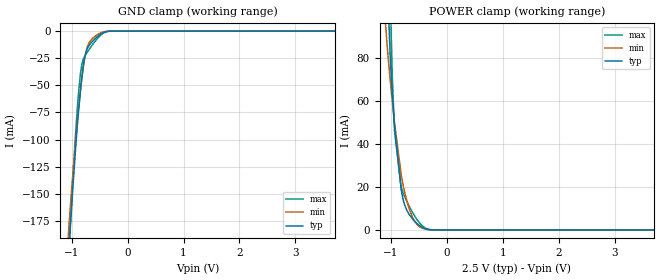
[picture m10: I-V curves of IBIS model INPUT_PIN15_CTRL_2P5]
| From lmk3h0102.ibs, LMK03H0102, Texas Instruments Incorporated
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[Model]   INPUT_PIN15_CTRL_2P5
Model_type   Input
Vinl = 0.4
Vinh = 1.625
|   typ   min   max
C_comp   0.7pF   0.5pF   0.9pF
[Voltage Range]   2.5   2.375   2.625
[Temperature Range]   45   125   -40
[Power Clamp Reference]   2.5   2.375   2.625
[GND Clamp Reference]   0   0   0
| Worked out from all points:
|   GND clamp passes 1 mA (typ) near -0.41 V on its own axis
|   POWER clamp passes 1 mA (typ) near -0.42 V on its own axis
[GND Clamp]
|   Voltage   I(typ)   I(min)   I(max)
-3.3V     -2.474A    -2.191A    -2.782A
-1.132V   -277.9mA   -243.6mA   -280mA
-1.043V   -198.1mA   -176.1mA   -194.8mA
-1.033V   -189.6mA   -169mA     -185.7mA
-1.013V   -173mA     -155.2mA   -167.6mA
-904.2mV  -91.28mA   -86.97mA   -75.43mA
-844.8mV  -56.1mA    -55.89mA   -39.89mA
-815.1mV  -41.69mA   -42.5mA    -30.02mA
-765.6mV  -24.25mA   -24.86mA   -23.17mA
-706.2mV  -14.74mA   -12.92mA   -18.37mA
-468.6mV  -2.382mA   -1.374mA   -3.243mA
6.6V      0A         0A         0A
[POWER Clamp]
|   Voltage   I(typ)   I(min)   I(max)
-3.3V     4.352A     3.467A     5.482A
-1.102V   157.7mA    98.45mA    260.3mA
-1.073V   126.7mA    87.91mA    205.9mA
-1.043V   101.6mA    78.59mA    156.2mA
-1.003V   76.72mA    67.34mA    101.2mA
-973.5mV  62.87mA    59.5mA     70.98mA
-933.9mV  48.26mA    49.68mA    45.87mA
-815.1mV  18.76mA    25.75mA    19.76mA
-745.8mV  11.11mA    16.79mA    15.13mA
-617.1mV  5.304mA    6.136mA    8.365mA
-419.1mV  966.3uA    632.5uA    1.565mA
6.6V      0A         0A         0A
